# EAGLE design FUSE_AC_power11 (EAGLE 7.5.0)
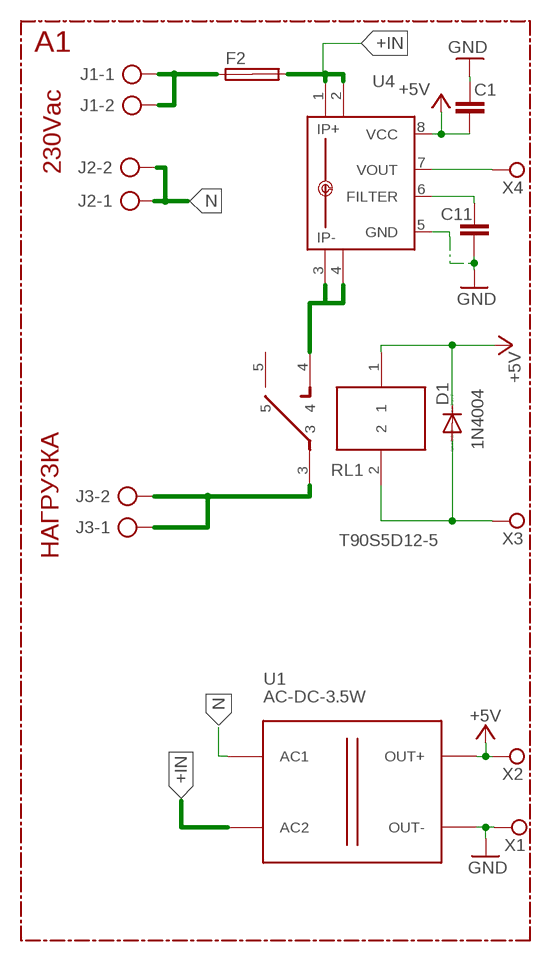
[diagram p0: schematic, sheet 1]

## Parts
C1  C-EUC0805  [C0805]
C11  C-EUC0805  [C0805]
D1  1N4004  [DO41-10]
F2  SHK20L  [SHK20L]
J1  AK300/2  [AK300/2]
J2  AK300/2  [AK300/2]
J3  AK300/2  [AK300/2]
RL1  T90S5D12-5  T9AS1D12  [T9A]
U1  AC-DC-3.5W  [AC-DC-3.5W]
U4  ACS712ELCTR-20A-T  [SO8]
X1  TPPAD1-20  [P1-20]
X2  TPPAD1-20  [P1-20]
X3  TPPAD1-20  [P1-20]
X4  TPPAD1-20  [P1-20]

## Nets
+5V: C1.1 D1.C RL1.1 U1.J2.3(OUT+) U4.8(VCC) X2.TP
+IN: F2.2A U1.J1.2(AC2) U4.1(IP+) U4.2(IP+1)
GND: C1.2 C11.1 U1.J2.1(OUT-) U4.5(GND) X1.TP
N: J2.1 J2.2 U1.J1.1(AC1)
N$1: U4.7(VOUT) X4.TP
N$16: F2.1A J1.1 J1.2
N$18: D1.A RL1.2 X3.TP
N$19: J3.1 J3.2 RL1.3
N$20: RL1.4 U4.3(IP-) U4.4(IP-1)
N$22: C11.2 U4.6(FILTER)
Unconnected: F2.1B F2.2B RL1.5

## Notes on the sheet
- А1
- 230Vac
- НАГРУЗКА

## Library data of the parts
C1 C11 = rcl:C-EU: CAPACITOR, European symbol
D1 = diode:1N4004: DIODE
F2 = fuse:SHK20L: FUSE HOLDER 5 x 20 mm, SH contact, SHH1 Schukat, E1073 Buerklin; OC_FARNELL: unknown; OC_NEWARK: unknown
J1-J3 = con-ptr500:AK300/2: CONNECTOR; OC_FARNELL: unknown; OC_NEWARK: unknown
RL1 = Mihail_soediniteli:T9AS1D12: RELAY 48V 30A Ambient temperature DC coil -55ºC to 85ºC
U1 = diy-modules:AC-DC-3.5W: AC/DC 3.5W Converter More details available here: https://www.itead.cc/wiki/AC-DC_Power_Module_5V_700mA Click here to find device on ebay.com
U4 = allegro:ACS712ELCTR-20A-T: Fully Integrated, Hall Effect-Based Linear Current Sensor with High Voltage Isolation and a Low-Resistance Current Conductor.
X1-X4 = testpad:TP: Test pad

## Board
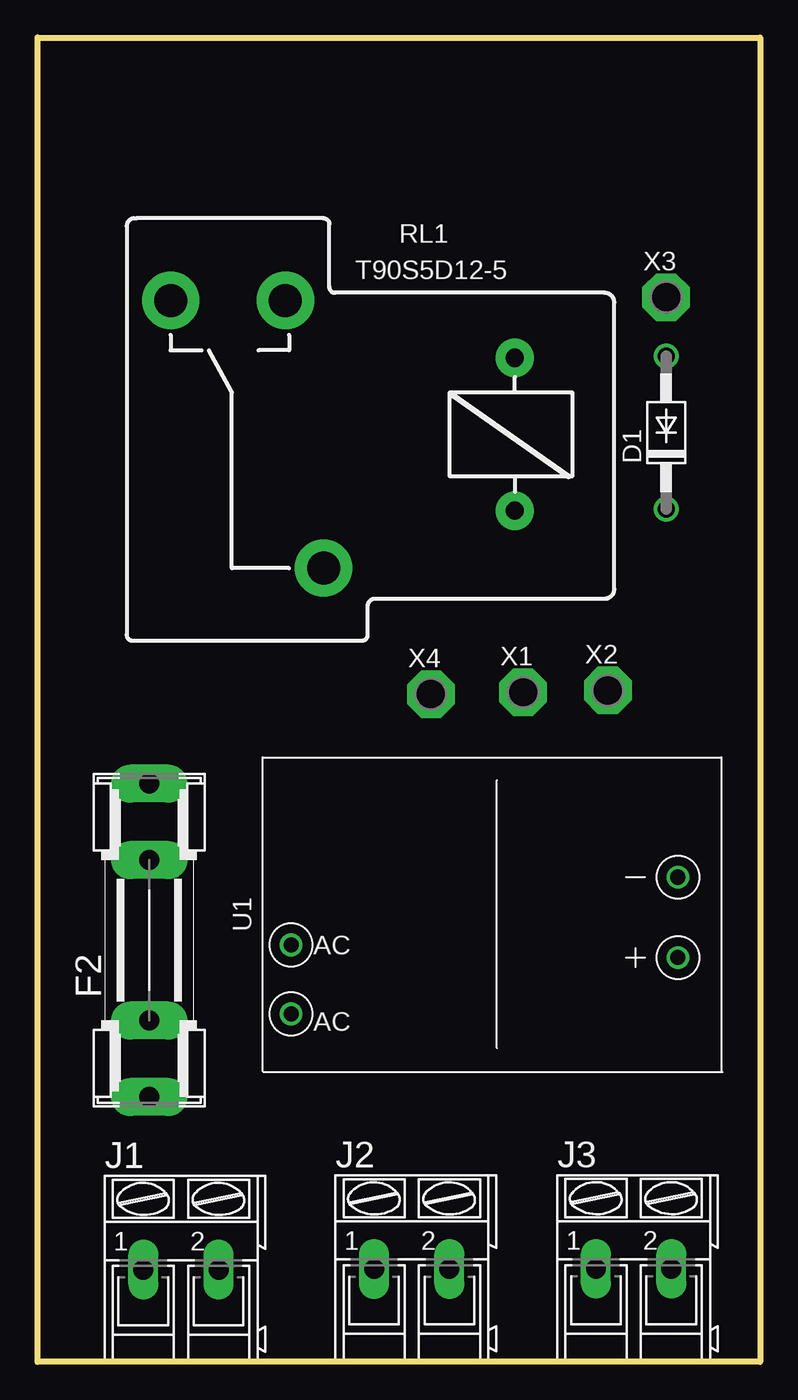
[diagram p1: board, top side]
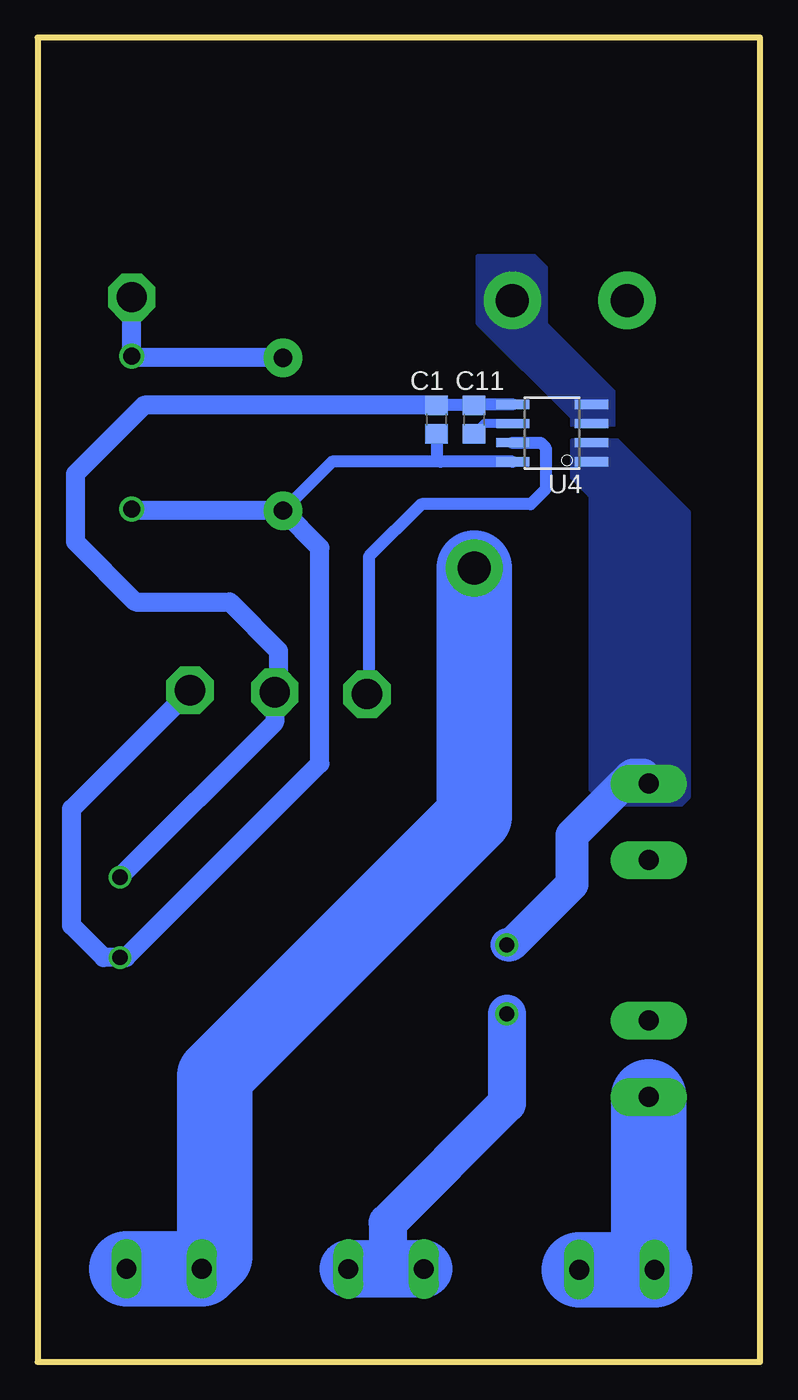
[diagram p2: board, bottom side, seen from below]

Size 48 x 88 mm. Coordinates in mm from the lower left corner, seen from the top.
Outline: 0,88 48,88 48,0 0,0 0,88
Copper layers (1*16): Top 0.035mm / dielectric 1.5mm / Bottom 0.035mm
Design rules "default": minimum track width 10mil, minimum drill 24mil, track to track 8mil, track to pad 8mil, pad to pad 8mil, via to via 8mil, smd to smd 8mil, copper to edge 40mil, drill to drill 8mil, minimum pad ring 10mil, minimum via ring 8mil, stop-mask expansion 4mil, vias tented up to drill 0mil, thermal gap 10mil

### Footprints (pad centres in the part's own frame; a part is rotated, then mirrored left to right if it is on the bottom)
C0805 = smd 1.3 x 1.5: 1 -0.95,0; 2 0.95,0
DO41-10 = drill 1.118: A 5.08,0; C -5.08,0
SHK20L = drill 1.321 pad 2.54 long: 1A -10.414,0; 1B -5.334,0; 2A 10.414,0; 2B 5.334,0
AK300/2 = drill 1.321 long: 1 -2.515,0; 2 2.489,0
T9A = drill 1.2 pad 2.54: 1 3.81,-12.7; 2 13.97,-12.7 | drill 2.2 pad 3.81: 3 0,0; 4 17.78,2.54; 5 17.78,10.16
AC-DC-3.5W = drill 1: J1.1 13.665,6.62; J1.2 13.665,2.04; J2.1 -12.03,-2.46; J2.3 -12.03,2.88
SO8 = smd 0.61 x 2.21: 1 0.635,-0.076; 2 1.905,-0.076; 3 3.175,-0.076; 4 4.445,-0.076; 5 4.445,5.156; 6 3.175,5.156; 7 1.905,5.156; 8 0.635,5.156
P1-20 = drill 2.007 pad 3.15 octagon: TP 0,0

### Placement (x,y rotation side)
C1  21.5,62.62 90 bottom
C11  19,62.62 270 bottom
D1  41.75,61.75 90 top
F2  7.41,28.02 90 top
J1  9.54,6.13 0 top
J2  24.86,6.17 0 top
J3  39.6,6.18 0 top
RL1  19,52.75 90 top
U1  30.5,29.75 180 top
U4  11.29,59.18 90 bottom
X1  32.25,44.5 0 top
X2  37.88,44.62 0 top
X3  41.75,70.75 0 top
X4  26.12,44.38 0 top

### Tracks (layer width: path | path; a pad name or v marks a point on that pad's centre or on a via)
+5V
  Bottom 0.813: U4.8 21.25,59.81 | 21.25,59.81 28.45,59.81 RL1.1 | C1.1 21.5,60.06 21.25,59.81
  Bottom 1.27: D1.C 41.64,56.56 RL1.1 29.25,54.11 29.25,39.75 42.13,26.87 U1.J2.3 43.62,26.87 45.75,29 45.75,36.75 X2.TP
+IN
  Bottom 2.184: U1.J1.2 16.54,27.71 12.5,31.75 12.5,35 8.5,39 7.75,39 7.75,38.77 F2.2A
  pour Bottom (no thermals): 12.5,61.25 9.5,61.25 4.75,56.5 4.75,37.5 5.25,37 10,37 10.5,37.5 10.75,37.5 11.25,38 11.25,57.5 12.5,58.75
GND
  Bottom 0.813: U4.5 18.95,63.62 C11.1 C1.2
  Bottom 1.27: U1.J2.1 32.25,42.49 X1.TP 32,44.75 32,47.25 35.25,50.5 41.5,50.5 45.5,54.5 45.5,59 40.92,63.58 C1.2
N
  Bottom 2.54: U1.J1.1 16.84,17.16 24.75,9.25 24.75,6.67 24.25,6.17
  Bottom 3.81: J2.1 24.25,6.17 J2.2
N$1
  Bottom 0.813: U4.7 14.59,61.09 14.25,60.75 14.25,58 15.25,57 22.5,57 26,53.5 26,44.5 X4.TP
N$16
  Bottom 3.81: 7.41,6.52 J1.1
  Bottom 5: J1.2 J1.1 | F2.1A 7.41,6.52
N$18
  Bottom 1.27: RL1.2 41.64,66.72 D1.A X3.TP
N$19
  Bottom 5: RL1.3 19,36.25 36.25,19 36.25,7.02 J3.1 J3.2
N$20
  pour Bottom (no thermals): 12.5,62.25 12.5,62.75 18.75,69 18.75,73.5 15,73.5 14.25,72.75 14.25,69 9.75,64.5 9.75,62.25
N$22
  Bottom 0.61: U4.6 18.32,62.36 C11.2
